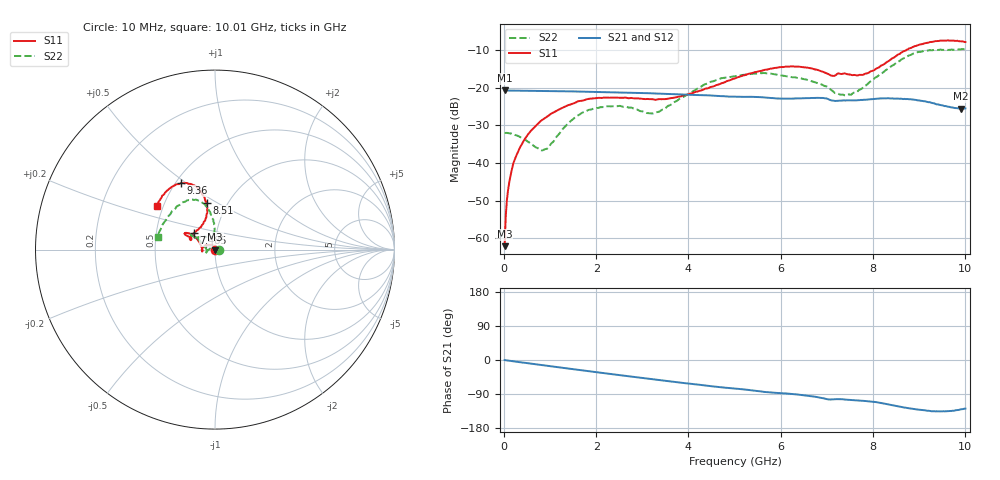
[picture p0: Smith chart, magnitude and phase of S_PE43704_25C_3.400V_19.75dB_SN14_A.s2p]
! Device ID: PE43704
! Dir: z:\PE43704\PE43704_Char_1_20130516\PE43704\AMB\3p400V\19p75dB
! Serial: 14
! Insertion: A
! Impedance: 50 ohm
! Temp: Amb
! VDD: 3.400V
! Attenuation Step: 19.75dB
! IDD: 1.141316e-01mA
#  Hz  S  RI  R  50
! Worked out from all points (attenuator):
!   401 points, 10 MHz to 10.01 GHz, reference 50 ohm
!   highest |S21| = -20.75 dB at 10 MHz (marker M1); lowest = -25.6 dB at 9.91 GHz (marker M2)
!   lowest |S11| = -62.1 dB at 10 MHz (marker M3), VSWR 1.00, Z = 50.1 + j0.0395 ohm
!   |S11| at or under -10 dB: start of sweep to 8.727 GHz
!   |S22| runs from -36.7 to -9.7 dB; largest |S21 - S12| = 0.0012
!   S11 on the Smith chart (normalised r, x): 10 MHz: 1.00, +0.00; 7.485 GHz: 0.78, +0.15; 8.51 GHz: 0.80, +0.45; 9.36 GHz: 0.53, +0.48; 10.01 GHz: 0.46, +0.27
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1e7  0.000676 0.000394  0.0918 -0.000285  0.0918 -0.000277  0.0249 0.000238
8.5e7  0.000739 0.00429  0.0917 -0.00239  0.0916 -0.0024  0.0248 0.00242
1.6e8  0.000309 0.00779  0.0914 -0.00443  0.0914 -0.0044  0.0241 0.00477
2.6e8  -0.00156 0.0122  0.0911 -0.00701  0.0911 -0.00696  0.022 0.00776
4.1e8  -0.00506 0.0183  0.0904 -0.011  0.0905 -0.0108  0.018 0.0114
8.85e8  -0.0267 0.029  0.0876 -0.0226  0.0876 -0.0225  -0.00445 0.0146
1.685e9  -0.0655 0.0143  0.079 -0.0406  0.079 -0.0406  -0.0452 -0.00944
2.36e9  -0.0736 -0.00486  0.0688 -0.0531  0.0688 -0.0531  -0.0516 -0.0242
3.36e9  -0.0704 -0.00186  0.0501 -0.0666  0.0502 -0.0665  -0.0478 0.00277
4.385e9  -0.0882 0.0416  0.0302 -0.0733  0.0305 -0.0732  -0.0946 0.0605
5.01e9  -0.1127 0.0705  0.0192 -0.0735  0.0193 -0.0736  -0.1219 0.0739
5.96e9  -0.161 0.0935  0.00356 -0.0717  0.00372 -0.0715  -0.1279 0.0737
6.685e9  -0.1612 0.0794  -0.00728 -0.0725  -0.00742 -0.0726  -0.1008 0.0675
7.11e9  -0.1308 0.0614  -0.0164 -0.0656  -0.0165 -0.0658  -0.0569 0.073
7.485e9  -0.1174 0.0939  -0.018 -0.0653  -0.018 -0.0655  -0.0221 0.0784
7.835e9  -0.0746 0.1339  -0.0217 -0.0655  -0.0214 -0.0659  -0.0035 0.1065
8.36e9  -0.0433 0.2253  -0.0337 -0.0637  -0.0337 -0.0641  -0.0159 0.1833
8.51e9  -0.0465 0.2605  -0.0373 -0.0613  -0.0372 -0.0612  -0.0284 0.2122
8.935e9  -0.0978 0.3453  -0.0444 -0.0525  -0.0443 -0.0523  -0.0944 0.2736
9.36e9  -0.1882 0.3708  -0.0435 -0.0425  -0.0438 -0.0427  -0.1864 0.26
9.91e9  -0.3057 0.2776  -0.0339 -0.0402  -0.0347 -0.04  -0.3037 0.1119
1.001e10  -0.3233 0.2436  -0.0328 -0.0417  -0.0335 -0.0422  -0.3184 0.0714
